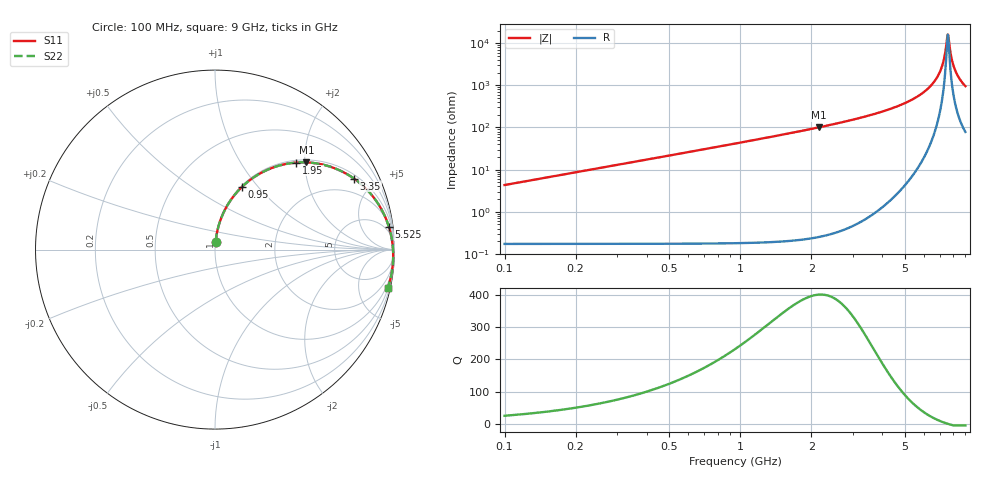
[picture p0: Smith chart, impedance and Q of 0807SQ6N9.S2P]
! Coilcraft 0807SQ-6N9 Air Core Inductor
! 06 March 2008
# MHZ S MA R 50
!Freq  MagS11  AngS11  MagS21  AngS21  MagS12  AngS12  MagS22  AngS22
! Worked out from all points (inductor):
!   357 points, 100 MHz to 9 GHz, reference 50 ohm
!   read as one part in series: L = 6.85 nH near 125 MHz
!   highest Q = 401 at 2.15 GHz (marker M1), where L = 7.45 nH
!   self-resonance near 7.575 GHz
!   S11 on the Smith chart (normalised r, x): 100 MHz: 1.00, +0.08; 950 MHz: 1.01, +0.82; 1.95 GHz: 1.05, +1.81; 3.35 GHz: 1.17, +3.82; 5.525 GHz: 3, +15; 9 GHz: 0.58, -9.14
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100  0.04237 85.2  0.9974 -2.5  0.9974 -2.5  0.04237 85.2
200  0.0845 83.9  0.9947 -5.0  0.9947 -5.0  0.08451 83.9
375  0.1573 80.1  0.9858 -9.3  0.9858 -9.3  0.1573 80.1
625  0.2576 74.3  0.9646 -15.4  0.9646 -15.4  0.2576 74.3
950  0.3785 66.9  0.9239 -22.9  0.9239 -22.9  0.3786 66.9
1600  0.5788 53.4  0.8138 -36.5  0.8138 -36.5  0.5789 53.4
1950  0.6629 47.0  0.747 -42.9  0.747 -42.9  0.6629 47.0
2150  0.704 43.6  0.7084 -46.2  0.7084 -46.2  0.7041 43.6
3075  0.8418 30.4  0.537 -59.5  0.537 -59.5  0.8419 30.4
3350  0.8698 27.0  0.4903 -62.7  0.4903 -62.7  0.8699 27.0
4550  0.9477 15.0  0.3116 -74.5  0.3116 -74.5  0.9478 15.0
5525  0.9777 7.3  0.1933 -81.7  0.1933 -81.7  0.9777 7.3
6050  0.9864 3.7  0.1377 -84.7  0.1377 -84.7  0.9865 3.7
6625  0.9918 0.0  0.08224 -86.7  0.08224 -86.7  0.9919 0.0
7050  0.9936 -2.5  0.04455 -85.6  0.04455 -85.6  0.9937 -2.5
7325  0.994 -4.0  0.02179 -78.8  0.02179 -78.8  0.9941 -4.0
7525  0.9939 -5.1  0.007666 -43.4  0.007666 -43.4  0.994 -5.1
7600  0.9938 -5.5  0.00625 5.8  0.00625 5.8  0.9939 -5.5
7825  0.9933 -6.7  0.01986 64.3  0.01986 64.3  0.9934 -6.7
8125  0.9922 -8.2  0.04188 72.2  0.04188 72.2  0.9923 -8.2
8500  0.9901 -10.1  0.06855 73.6  0.06855 73.6  0.9902 -10.1
9000  0.9864 -12.4  0.1021 72.9  0.1021 72.9  0.9865 -12.4
